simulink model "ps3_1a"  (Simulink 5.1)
settings: Solver=ode45  StartTime=0.0  StopTime=10.0  RelTol=1e-3
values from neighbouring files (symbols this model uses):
  a = [a -1*(1+m/100)]    [ps7_3_2.m]
  s = tf('s')    [ps7_3_2.m]    (also in ps4_2.m; ps7_1_2.m; ps4_3.m; ps2_3.m)
libraries: cstblocks x1

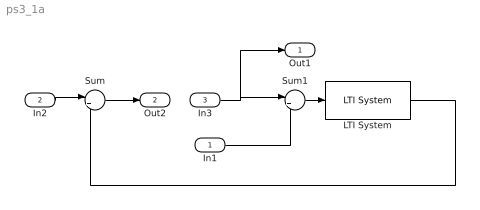
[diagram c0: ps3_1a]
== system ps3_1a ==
  In1 : Inport
  In2 : Inport  Port=2
  In3 : Inport  Port=3
  LTI System : cstblocks/LTI System  sys=1/(s^2-a^2)  IC=[]
  Sum : Sum  Inputs=|++
  Sum1 : Sum  Inputs=|++
  Out1 : Outport
  Out2 : Outport  Port=2
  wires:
  In2/1 -> Sum/1
  Sum/1 -> Out2/1
  In3/1 -> Sum1/1, Out1/1
  In1/1 -> Sum1/2
  Sum1/1 -> LTI System/1
  LTI System/1 -> Sum/2
